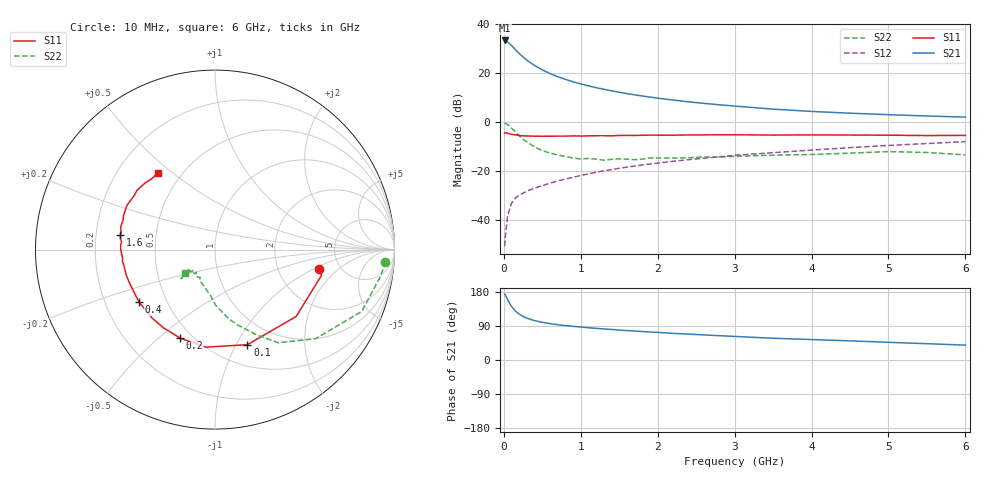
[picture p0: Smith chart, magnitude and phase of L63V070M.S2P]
!  INFINEON TECHNOLOGIES Small Signal Semiconductors
! BFR380L3 , Si-NPN RF-Transistor in TSLP-3-1
!  Vce=3 V,  Ic=70 mA
! Common Emitter S-Parameters:  07. March 2005
#  GHz  S  MA  R  50
! f  S11  S21  S12  S22
! GHz  Mag  Ang  Mag  Ang  Mag  Ang  Mag  Ang
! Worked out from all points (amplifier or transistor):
!   36 points, 10 MHz to 6 GHz, reference 50 ohm
!   highest |S21| = 33.3 dB at 10 MHz (marker M1)
!   |S21| within 3 dB of that: start of sweep to 127.7 MHz
!   unconditionally stable (mu >= 1): 1.307 GHz to 4.842 GHz
!   at 250 MHz: K = 0.54, MSG = 27.8 dB, |S12| = -29.1 dB
!   at 1.4 GHz: K = 1.01, MAG = 15.5 dB, |S12| = -19.5 dB
!   at 6 GHz: K = 0.97, MSG = 5.0 dB, |S12| = -8.0 dB
!   S11 on the Smith chart (normalised r, x): 10 MHz: 3.45, -1.17; 100 MHz: 0.72, -1.11; 200 MHz: 0.43, -0.59; 400 MHz: 0.35, -0.27; 1.6 GHz: 0.31, +0.07; 6 GHz: 0.37, +0.44
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0.01  0.5904 -10.8  46.45 173.9  0.0029 78.7  0.9511 -4.0
0.02  0.6103 -13.7  45.96 171.3  0.0047 79.0  0.9344 -9.1
0.05  0.5859 -39.5  43.33 158.3  0.0123 74.9  0.8874 -22.8
0.1  0.5596 -71.2  36.54 141.4  0.0219 63.7  0.7489 -41.5
0.15  0.5461 -95.4  30.21 129.1  0.0279 57.6  0.6276 -55.8
0.2  0.53 -111.4  25.1 120.9  0.032 55.6  0.5253 -64.3
0.25  0.5219 -123.4  21.31 115.0  0.0352 53.8  0.4417 -72.8
0.3  0.518 -132.4  18.3 110.4  0.0388 54.7  0.3934 -78.8
0.4  0.5141 -145.6  14.28 103.8  0.0446 55.9  0.3091 -89.4
0.5  0.5098 -154.0  11.65 99.5  0.0502 58.0  0.2598 -95.0
0.6  0.5121 -160.1  9.758 96.0  0.0561 59.6  0.2328 -101.1
0.7  0.5148 -164.5  8.455 93.3  0.0627 61.5  0.2114 -107.4
0.9  0.5196 -173.0  6.62 88.8  0.0742 64.1  0.1837 -117.5
1.1  0.5215 -177.8  5.476 85.1  0.0873 65.5  0.1806 -122.4
1.3  0.5262 177.1  4.669 81.9  0.1008 66.4  0.1659 -129.9
1.6  0.534 171.3  3.812 77.6  0.12 67.1  0.1736 -136.7
2.2  0.538 162.4  2.813 70.4  0.1576 67.3  0.183 -137.7
2.8  0.5488 154.1  2.25 64.2  0.1945 67.1  0.1927 -143.3
3.5  0.5413 146.0  1.834 57.4  0.2364 64.7  0.2104 -141.3
4.5  0.5419 140.1  1.515 50.5  0.2996 62.8  0.231 -140.1
5.5  0.5293 132.0  1.328 43.0  0.3634 58.8  0.2383 -139.7
6  0.5328 126.9  1.261 39.3  0.397 56.6  0.213 -142.0
